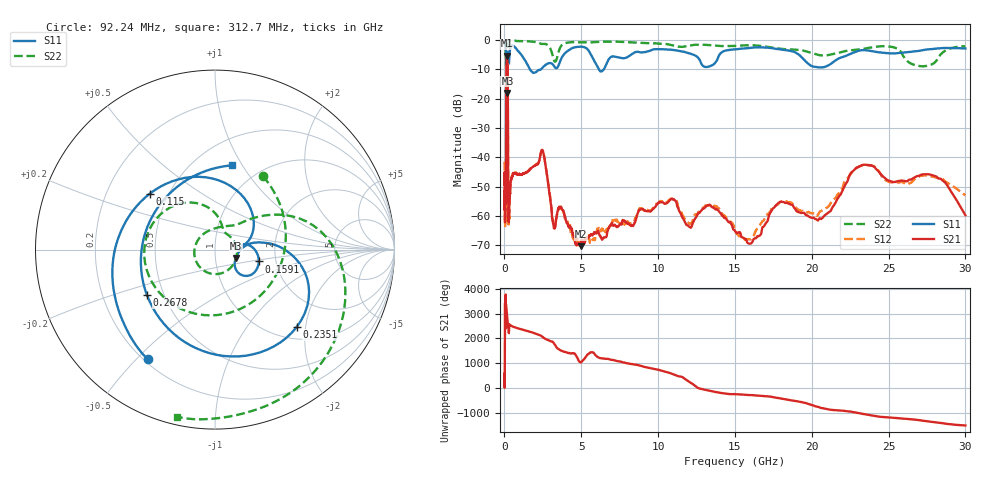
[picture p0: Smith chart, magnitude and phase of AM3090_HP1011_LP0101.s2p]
! Date/Time: Thu, Feb 28, 2019 2:05 PM
! Network Analyzer: Agilent Technologies E8364B Rev: A.07.50.67
! Sweep from 0.010 to 30.000 GHz, 1601 Points, Sweep Type: LOG
! Power Supply: 5.023 V, 0.002 A
# Hz S DB R 50
!freq MagS11 AngS11 MagS21 AngS21 MagS12 AngS12 MagS22 AngS22
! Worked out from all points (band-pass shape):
!   1601 points, 10 MHz to 30 GHz, reference 50 ohm
!   highest |S21| = -5.39 dB at 164 MHz (marker M1); lowest = -70.3 dB at 4.952 GHz (marker M2)
!   |S21| within 3 dB of the highest: 130.2 MHz to 205.5 MHz (75.3 MHz wide, 44.9 % of centre)
!   lowest |S11| = -18.1 dB at 192.5 MHz (marker M3), VSWR 1.28, Z = 62.7 - j6.03 ohm
!   |S11| at or under -10 dB: 125.2 MHz to 213.5 MHz (88.33 MHz wide, 52.2 % of centre); 1.657 GHz to 2.376 GHz (719.5 MHz wide, 35.7 % of centre); 6.146 GHz to 6.467 GHz (320.4 MHz wide, 5.08 % of centre)
!   |S22| runs from -19.4 to -0.2 dB; largest |S21 - S12| = 0.011
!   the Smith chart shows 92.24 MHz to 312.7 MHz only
!   S11 on the Smith chart (normalised r, x): 92.24 MHz: 0.21, -0.54; 115 MHz: 0.39, +0.32; 159.1 MHz: 1.63, -0.23; 235.1 MHz: 1.26, -1.79; 267.8 MHz: 0.40, -0.26; 312.7 MHz: 0.74, +0.90
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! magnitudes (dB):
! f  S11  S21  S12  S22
! 10 MHz  -0.3  -49.4  -41.5  -0.6
! 38.04 MHz  -0.4  -60.6  -61.7  -1.3
! 49.84 MHz  -0.7  -50.8  -48.3  -1.4
! 92.24 MHz  -2.9  -55.1  -54.9  -6.2
! 115 MHz  -6.4  -22.6  -22.7  -8.1
! 144.7 MHz  -14.8  -5.8  -5.8  -19.2
! 159.1 MHz  -12.0  -5.4  -5.4  -17.6
! 164 MHz  -11.8  -5.4  -5.4  -17.3
! 192.5 MHz  -18.1  -6.3  -6.3  -19.1
! 214.9 MHz  -9.5  -12.8  -12.8  -11.5
! 235.1 MHz  -4.1  -40.3  -39.9  -2.7
! 267.8 MHz  -6.8  -60.0  -61.4  -0.8
! 312.7 MHz  -6.4  -57.3  -60.5  -0.4
! 550.5 MHz  -2.0  -45.8  -45.4  -0.2
! 2.084 GHz  -10.8  -42.5  -42.3  -0.8
! 2.495 GHz  -9.4  -37.8  -37.7  -1.3
! 3.204 GHz  -8.7  -63.6  -62.6  -6.7
! 4.952 GHz  -2.3  -70.3  -69.4  -0.8
! 7.926 GHz  -6.0  -62.3  -62.4  -0.7
! 16.05 GHz  -2.7  -69.4  -67.9  -1.8
! 23.48 GHz  -3.5  -42.5  -42.7  -2.9
! 30 GHz  -2.9  -59.7  -53.0  -2.2
